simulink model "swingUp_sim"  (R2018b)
settings: Solver=ode4  StartTime=0.0  StopTime=T+Tstb  FixedStep=1e-3  MaxStep=1e-3  RelTol=1e-3  AbsTol=1e-6
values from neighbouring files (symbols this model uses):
  b_0 = (bp_0 + bn_0) / 2    [mainSkript_provedeniSimulaceSwingUp.m]    (also in mainSkript_rovniceSystemu.m = (params.bp_0 + params.bn_0) / 2; mainSkript_overeniRovnic.m = 0; mainSkript_simulaceLQG.m = (bn_0 + bp_0) / 2; mainSkript_LQGexperiment.m = (bn_0 + bp_0) / 2)
  b_1 = params.b_1    [mainSkript_provedeniSimulaceSwingUp.m]    (also in mainSkript_rovniceSystemu.m; mainSkript_overeniRovnic.m; mainSkript_kyvadlaNajednouOdhad.m; mainSkript_simulaceLQG.m)
  b_2 = params.b_2    [mainSkript_provedeniSimulaceSwingUp.m]    (also in mainSkript_rovniceSystemu.m; mainSkript_overeniRovnic.m; mainSkript_kyvadlaNajednouOdhad.m; mainSkript_simulaceLQG.m)
  g = 9.81    [mainSkript_provedeniSimulaceSwingUp.m]    (also in mainSkript_rovniceSystemu.m; mainSkript_overeniRovnic.m; mainSkript_estimaceVozik.m; mainSkript_odhadKyvadlaZvlast.m)
  I_1 = params.I_1    [mainSkript_provedeniSimulaceSwingUp.m]    (also in mainSkript_rovniceSystemu.m; mainSkript_overeniRovnic.m; mainSkript_kyvadlaNajednouOdhad.m; mainSkript_simulaceLQG.m)
  I_2 = params.I_2    [mainSkript_provedeniSimulaceSwingUp.m]    (also in mainSkript_rovniceSystemu.m; mainSkript_overeniRovnic.m; mainSkript_kyvadlaNajednouOdhad.m; mainSkript_simulaceLQG.m)
  K = lqr(sysd, Q_lqr, R_lqr)    [mainSkript_provedeniSimulaceSwingUp.m]    (also in makeFBL.m = [0; -d_2*g*sin(th_1); -d_3*g*sin(th_2)]; mainSkript_simulaceLQG.m = lqr(sysd, Qk, Rk); mainSkript_LQGexperiment.m = lqr(sysd, Q, R); mainSkript_LQGexperiment_integral.m = lqr(sysd, Q, R))
  K1 = [K1(1 : idxL-rez); K1(idxL : idxH); K1(idxH+rez : end)]    [mainSkript_provedeniSimulaceSwingUp.m]
  K2 = [K2(1 : idxL-rez); K2(idxL : idxH); K2(idxH+rez : end)]    [mainSkript_provedeniSimulaceSwingUp.m]
  K3 = [K3(1 : idxL-rez); K3(idxL : idxH); K3(idxH+rez : end)]    [mainSkript_provedeniSimulaceSwingUp.m]
  K4 = [K4(1 : idxL-rez); K4(idxL : idxH); K4(idxH+rez : end)]    [mainSkript_provedeniSimulaceSwingUp.m]
  K5 = [K5(1 : idxL-rez); K5(idxL : idxH); K5(idxH+rez : end)]    [mainSkript_provedeniSimulaceSwingUp.m]
  K6 = [K6(1 : idxL-rez); K6(idxL : idxH); K6(idxH+rez : end)]    [mainSkript_provedeniSimulaceSwingUp.m]
  Ki = [Ki(1 : idxL-rez); Ki(idxL : idxH); Ki(idxH+rez : end)]    [mainSkript_provedeniSimulaceSwingUp.m]
  L_1 = params.L_1    [mainSkript_provedeniSimulaceSwingUp.m]    (also in mainSkript_rovniceSystemu.m; mainSkript_overeniRovnic.m; odhadovane_parametry.m = 0.228; mainSkript_kyvadlaNajednouOdhad.m)
  l_1 = params.l_1    [mainSkript_provedeniSimulaceSwingUp.m]    (also in mainSkript_rovniceSystemu.m; mainSkript_overeniRovnic.m; odhadovane_parametry.m = 0.134; mainSkript_kyvadlaNajednouOdhad.m)
  l_2 = params.l_2    [mainSkript_provedeniSimulaceSwingUp.m]    (also in mainSkript_rovniceSystemu.m; mainSkript_overeniRovnic.m; odhadovane_parametry.m = 0.112; mainSkript_kyvadlaNajednouOdhad.m)
  m_0 = params.m_0    [mainSkript_provedeniSimulaceSwingUp.m]    (also in mainSkript_rovniceSystemu.m; mainSkript_overeniRovnic.m; mainSkript_simulaceLQG.m; mainSkript_LQGexperiment.m)
  m_1 = params.m_1    [mainSkript_provedeniSimulaceSwingUp.m]    (also in mainSkript_rovniceSystemu.m; mainSkript_overeniRovnic.m; mainSkript_kyvadlaNajednouOdhad.m; mainSkript_simulaceLQG.m)
  m_2 = params.m_2    [mainSkript_provedeniSimulaceSwingUp.m]    (also in mainSkript_rovniceSystemu.m; mainSkript_overeniRovnic.m; mainSkript_kyvadlaNajednouOdhad.m; mainSkript_simulaceLQG.m)
  q_0 = [theta0(1) theta1(1) theta2(1) dtheta0(1) dtheta1(1) dtheta2(1)]    [mainSkript_provedeniSimulaceSwingUp.m]    (also in mainSkript_kyvadlaNajednouOdhad.m = cell(1, k); mainSkript_simulaceLQG.m = [0 th1_0 th2_0 0 dth1_0 dth2_0]; mainSkript_LQGexperiment.m = zeros(6,1); mainSkript_LQGexperiment_integral.m = zeros(6,1))
  Q_stab = diag([0.1 6e-3 6e-3 1.2 0.6 0.6])    [mainSkript_provedeniSimulaceSwingUp.m]
  Q_swing = diag([10 10 10 100 100 100])    [mainSkript_provedeniSimulaceSwingUp.m]
  R_stab = diag([0.1 0.5 0.5])    [mainSkript_provedeniSimulaceSwingUp.m]
  R_swing = diag([1 1 1])    [mainSkript_provedeniSimulaceSwingUp.m]
  t_FB = [t_FB(1 : idxL-rez); t_FB(idxL : idxH); t_FB(idxH+rez : end)]    [mainSkript_provedeniSimulaceSwingUp.m]
  Ts = 1e-3    (= 0.001)    [mainSkript_provedeniSimulaceSwingUp.m]    (also in mainSkript_rovniceSystemu.m; mainSkript_simulaceLQG.m; mainSkript_LQGexperiment.m; mainSkript_LQGexperiment_integral.m)
undefined symbols (not defined in the file or in its folder): DiscIntNeverNeededParam
libraries: simulink x5, sharedTrackingLibrary x1
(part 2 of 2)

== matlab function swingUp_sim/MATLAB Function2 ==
function dx = PohybovaRceDIP_basic(y, u, g, m_0, m_1, m_2, I_1, I_2, l_1, l_2, L_1, b_0, b_1, b_2)
%PohybovaRceDIP_basic: Pohybova rovnice dvojiteho kyvadla

dx = zeros(6, 1); % definovani sloupcoveho vektoru derivaci stavu 

dx(1) = conj(y(4)); 
dx(2) = conj(y(5)); 
dx(3) = conj(y(6)); 
dx(4) = conj(y(6))*((b_2*(L_1^2*l_2*m_2^2*cos(y(3)) + I_1*l_2*m_2*cos(y(3)) - L_1^2*l_2*m_2^2*cos(y(2) - y(3))*cos(y(2)) + l_1^2*l_2*m_1*m_2*cos(y(3)) - L_1*l_1*l_2*m_1*m_2*cos(y(2) - y(3))*cos(y(2))))/(I_2*L_1^2*m_2^2 + I_2*l_1^2*m_1^2 + I_1*l_2^2*m_2^2 + I_1*I_2*m_0 + I_1*I_2*m_1 + I_1*I_2*m_2 + L_1^2*l_2^2*m_2^3 + L_1^2*l_2^2*m_0*m_2^2 + L_1^2*l_2^2*m_1*m_2^2 - L_1^2*l_2^2*m_2^3*cos(y(2) - y(3))^2 + I_2*L_1^2*m_0*m_2 + I_2*L_1^2*m_1*m_2 + l_1^2*l_2^2*m_1*m_2^2 + l_1^2*l_2^2*m_1^2*m_2 + I_2*l_1^2*m_0*m_1 + I_1*l_2^2*m_0*m_2 + I_1*l_2^2*m_1*m_2 + I_2*l_1^2*m_1*m_2 - I_2*L_1^2*m_2^2*cos(y(2))^2 - I_2*l_1^2*m_1^2*cos(y(2))^2 - I_1*l_2^2*m_2^2*cos(y(3))^2 - L_1^2*l_2^2*m_2^3*cos(y(2))^2 - L_1^2*l_2^2*m_2^3*cos(y(3))^2 + l_1^2*l_2^2*m_0*m_1*m_2 - l_1^2*l_2^2*m_1^2*m_2*cos(y(2))^2 - l_1^2*l_2^2*m_1*m_2^2*cos(y(3))^2 - L_1^2*l_2^2*m_0*m_2^2*cos(y(2) - y(3))^2 - L_1^2*l_2^2*m_1*m_2^2*cos(y(2) - y(3))^2 - 2*L_1*l_1*l_2^2*m_1*m_2^2*cos(y(2))^2 + 2*L_1^2*l_2^2*m_2^3*cos(y(2) - y(3))*cos(y(2))*cos(y(3)) - 2*I_2*L_1*l_1*m_1*m_2*cos(y(2))^2 + 2*L_1*l_1*l_2^2*m_1*m_2^2*cos(y(2) - y(3))*cos(y(2))*cos(y(3))) - ((b_2 - L_1*l_2*m_2*sin(y(2) - y(3))*y(6))*(L_1*l_2^2*m_2^2*cos(y(2)) + I_2*L_1*m_2*cos(y(2)) + I_2*l_1*m_1*cos(y(2)) - L_1*l_2^2*m_2^2*cos(y(2) - y(3))*cos(y(3)) + l_1*l_2^2*m_1*m_2*cos(y(2))))/(I_2*L_1^2*m_2^2 + I_2*l_1^2*m_1^2 + I_1*l_2^2*m_2^2 + I_1*I_2*m_0 + I_1*I_2*m_1 + I_1*I_2*m_2 + L_1^2*l_2^2*m_2^3 + L_1^2*l_2^2*m_0*m_2^2 + L_1^2*l_2^2*m_1*m_2^2 - L_1^2*l_2^2*m_2^3*cos(y(2) - y(3))^2 + I_2*L_1^2*m_0*m_2 + I_2*L_1^2*m_1*m_2 + l_1^2*l_2^2*m_1*m_2^2 + l_1^2*l_2^2*m_1^2*m_2 + I_2*l_1^2*m_0*m_1 + I_1*l_2^2*m_0*m_2 + I_1*l_2^2*m_1*m_2 + I_2*l_1^2*m_1*m_2 - I_2*L_1^2*m_2^2*cos(y(2))^2 - I_2*l_1^2*m_1^2*cos(y(2))^2 - I_1*l_2^2*m_2^2*cos(y(3))^2 - L_1^2*l_2^2*m_2^3*cos(y(2))^2 - L_1^2*l_2^2*m_2^3*cos(y(3))^2 + l_1^2*l_2^2*m_0*m_1*m_2 - l_1^2*l_2^2*m_1^2*m_2*cos(y(2))^2 - l_1^2*l_2^2*m_1*m_2^2*cos(y(3))^2 - L_1^2*l_2^2*m_0*m_2^2*cos(y(2) - y(3))^2 - L_1^2*l_2^2*m_1*m_2^2*cos(y(2) - y(3))^2 - 2*L_1*l_1*l_2^2*m_1*m_2^2*cos(y(2))^2 + 2*L_1^2*l_2^2*m_2^3*cos(y(2) - y(3))*cos(y(2))*cos(y(3)) - 2*I_2*L_1*l_1*m_1*m_2*cos(y(2))^2 + 2*L_1*l_1*l_2^2*m_1*m_2^2*cos(y(2) - y(3))*cos(y(2))*cos(y(3))) + (l_2*m_2*y(6)*sin(y(3))*(I_1*I_2 + L_1^2*l_2^2*m_2^2 + I_2*L_1^2*m_2 + I_2*l_1^2*m_1 + I_1*l_2^2*m_2 - L_1^2*l_2^2*m_2^2*cos(y(2) - y(3))^2 + l_1^2*l_2^2*m_1*m_2))/(I_2*L_1^2*m_2^2 + I_2*l_1^2*m_1^2 + I_1*l_2^2*m_2^2 + I_1*I_2*m_0 + I_1*I_2*m_1 + I_1*I_2*m_2 + L_1^2*l_2^2*m_2^3 + L_1^2*l_2^2*m_0*m_2^2 + L_1^2*l_2^2*m_1*m_2^2 - L_1^2*l_2^2*m_2^3*cos(y(2) - y(3))^2 + I_2*L_1^2*m_0*m_2 + I_2*L_1^2*m_1*m_2 + l_1^2*l_2^2*m_1*m_2^2 + l_1^2*l_2^2*m_1^2*m_2 + I_2*l_1^2*m_0*m_1 + I_1*l_2^2*m_0*m_2 + I_1*l_2^2*m_1*m_2 + I_2*l_1^2*m_1*m_2 - I_2*L_1^2*m_2^2*cos(y(2))^2 - I_2*l_1^2*m_1^2*cos(y(2))^2 - I_1*l_2^2*m_2^2*cos(y(3))^2 - L_1^2*l_2^2*m_2^3*cos(y(2))^2 - L_1^2*l_2^2*m_2^3*cos(y(3))^2 + l_1^2*l_2^2*m_0*m_1*m_2 - l_1^2*l_2^2*m_1^2*m_2*cos(y(2))^2 - l_1^2*l_2^2*m_1*m_2^2*cos(y(3))^2 - L_1^2*l_2^2*m_0*m_2^2*cos(y(2) - y(3))^2 - L_1^2*l_2^2*m_1*m_2^2*cos(y(2) - y(3))^2 - 2*L_1*l_1*l_2^2*m_1*m_2^2*cos(y(2))^2 + 2*L_1^2*l_2^2*m_2^3*cos(y(2) - y(3))*cos(y(2))*cos(y(3)) - 2*I_2*L_1*l_1*m_1*m_2*cos(y(2))^2 + 2*L_1*l_1*l_2^2*m_1*m_2^2*cos(y(2) - y(3))*cos(y(2))*cos(y(3)))) + conj(y(5))*(((b_1 + b_2)*(L_1*l_2^2*m_2^2*cos(y(2)) + I_2*L_1*m_2*cos(y(2)) + I_2*l_1*m_1*cos(y(2)) - L_1*l_2^2*m_2^2*cos(y(2) - y(3))*cos(y(3)) + l_1*l_2^2*m_1*m_2*cos(y(2))))/(I_2*L_1^2*m_2^2 + I_2*l_1^2*m_1^2 + I_1*l_2^2*m_2^2 + I_1*I_2*m_0 + I_1*I_2*m_1 + I_1*I_2*m_2 + L_1^2*l_2^2*m_2^3 + L_1^2*l_2^2*m_0*m_2^2 + L_1^2*l_2^2*m_1*m_2^2 - L_1^2*l_2^2*m_2^3*cos(y(2) - y(3))^2 + I_2*L_1^2*m_0*m_2 + I_2*L_1^2*m_1*m_2 + l_1^2*l_2^2*m_1*m_2^2 + l_1^2*l_2^2*m_1^2*m_2 + I_2*l_1^2*m_0*m_1 + I_1*l_2^2*m_0*m_2 + I_1*l_2^2*m_1*m_2 + I_2*l_1^2*m_1*m_2 - I_2*L_1^2*m_2^2*cos(y(2))^2 - I_2*l_1^2*m_1^2*cos(y(2))^2 - I_1*l_2^2*m_2^2*cos(y(3))^2 - L_1^2*l_2^2*m_2^3*cos(y(2))^2 - L_1^2*l_2^2*m_2^3*cos(y(3))^2 + l_1^2*l_2^2*m_0*m_1*m_2 - l_1^2*l_2^2*m_1^2*m_2*cos(y(2))^2 - l_1^2*l_2^2*m_1*m_2^2*cos(y(3))^2 - L_1^2*l_2^2*m_0*m_2^2*cos(y(2) - y(3))^2 - L_1^2*l_2^2*m_1*m_2^2*cos(y(2) - y(3))^2 - 2*L_1*l_1*l_2^2*m_1*m_2^2*cos(y(2))^2 + 2*L_1^2*l_2^2*m_2^3*cos(y(2) - y(3))*cos(y(2))*cos(y(3)) - 2*I_2*L_1*l_1*m_1*m_2*cos(y(2))^2 + 2*L_1*l_1*l_2^2*m_1*m_2^2*cos(y(2) - y(3))*cos(y(2))*cos(y(3))) - ((b_2 + L_1*l_2*m_2*sin(y(2) - y(3))*y(5))*(L_1^2*l_2*m_2^2*cos(y(3)) + I_1*l_2*m_2*cos(y(3)) - L_1^2*l_2*m_2^2*cos(y(2) - y(3))*cos(y(2)) + l_1^2*l_2*m_1*m_2*cos(y(3)) - L_1*l_1*l_2*m_1*m_2*cos(y(2) - y(3))*cos(y(2))))/(I_2*L_1^2*m_2^2 + I_2*l_1^2*m_1^2 + I_1*l_2^2*m_2^2 + I_1*I_2*m_0 + I_1*I_2*m_1 + I_1*I_2*m_2 + L_1^2*l_2^2*m_2^3 + L_1^2*l_2^2*m_0*m_2^2 + L_1^2*l_2^2*m_1*m_2^2 - L_1^2*l_2^2*m_2^3*cos(y(2) - y(3))^2 + I_2*L_1^2*m_0*m_2 + I_2*L_1^2*m_1*m_2 + l_1^2*l_2^2*m_1*m_2^2 + l_1^2*l_2^2*m_1^2*m_2 + I_2*l_1^2*m_0*m_1 + I_1*l_2^2*m_0*m_2 + I_1*l_2^2*m_1*m_2 + I_2*l_1^2*m_1*m_2 - I_2*L_1^2*m_2^2*cos(y(2))^2 - I_2*l_1^2*m_1^2*cos(y(2))^2 - I_1*l_2^2*m_2^2*cos(y(3))^2 - L_1^2*l_2^2*m_2^3*cos(y(2))^2 - L_1^2*l_2^2*m_2^3*cos(y(3))^2 + l_1^2*l_2^2*m_0*m_1*m_2 - l_1^2*l_2^2*m_1^2*m_2*cos(y(2))^2 - l_1^2*l_2^2*m_1*m_2^2*cos(y(3))^2 - L_1^2*l_2^2*m_0*m_2^2*cos(y(2) - y(3))^2 - L_1^2*l_2^2*m_1*m_2^2*cos(y(2) - y(3))^2 - 2*L_1*l_1*l_2^2*m_1*m_2^2*cos(y(2))^2 + 2*L_1^2*l_2^2*m_2^3*cos(y(2) - y(3))*cos(y(2))*cos(y(3)) - 2*I_2*L_1*l_1*m_1*m_2*cos(y(2))^2 + 2*L_1*l_1*l_2^2*m_1*m_2^2*cos(y(2) - y(3))*cos(y(2))*cos(y(3))) + (y(5)*sin(y(2))*(L_1*m_2 + l_1*m_1)*(I_1*I_2 + L_1^2*l_2^2*m_2^2 + I_2*L_1^2*m_2 + I_2*l_1^2*m_1 + I_1*l_2^2*m_2 - L_1^2*l_2^2*m_2^2*cos(y(2) - y(3))^2 + l_1^2*l_2^2*m_1*m_2))/(I_2*L_1^2*m_2^2 + I_2*l_1^2*m_1^2 + I_1*l_2^2*m_2^2 + I_1*I_2*m_0 + I_1*I_2*m_1 + I_1*I_2*m_2 + L_1^2*l_2^2*m_2^3 + L_1^2*l_2^2*m_0*m_2^2 + L_1^2*l_2^2*m_1*m_2^2 - L_1^2*l_2^2*m_2^3*cos(y(2) - y(3))^2 + I_2*L_1^2*m_0*m_2 + I_2*L_1^2*m_1*m_2 + l_1^2*l_2^2*m_1*m_2^2 + l_1^2*l_2^2*m_1^2*m_2 + I_2*l_1^2*m_0*m_1 + I_1*l_2^2*m_0*m_2 + I_1*l_2^2*m_1*m_2 + I_2*l_1^2*m_1*m_2 - I_2*L_1^2*m_2^2*cos(y(2))^2 - I_2*l_1^2*m_1^2*cos(y(2))^2 - I_1*l_2^2*m_2^2*cos(y(3))^2 - L_1^2*l_2^2*m_2^3*cos(y(2))^2 - L_1^2*l_2^2*m_2^3*cos(y(3))^2 + l_1^2*l_2^2*m_0*m_1*m_2 - l_1^2*l_2^2*m_1^2*m_2*cos(y(2))^2 - l_1^2*l_2^2*m_1*m_2^2*cos(y(3))^2 - L_1^2*l_2^2*m_0*m_2^2*cos(y(2) - y(3))^2 - L_1^2*l_2^2*m_1*m_2^2*cos(y(2) - y(3))^2 - 2*L_1*l_1*l_2^2*m_1*m_2^2*cos(y(2))^2 + 2*L_1^2*l_2^2*m_2^3*cos(y(2) - y(3))*cos(y(2))*cos(y(3)) - 2*I_2*L_1*l_1*m_1*m_2*cos(y(2))^2 + 2*L_1*l_1*l_2^2*m_1*m_2^2*cos(y(2) - y(3))*cos(y(2))*cos(y(3)))) + (u*(I_1*I_2 + L_1^2*l_2^2*m_2^2 + I_2*L_1^2*m_2 + I_2*l_1^2*m_1 + I_1*l_2^2*m_2 - L_1^2*l_2^2*m_2^2*cos(y(2) - y(3))^2 + l_1^2*l_2^2*m_1*m_2))/(I_2*L_1^2*m_2^2 + I_2*l_1^2*m_1^2 + I_1*l_2^2*m_2^2 + I_1*I_2*m_0 + I_1*I_2*m_1 + I_1*I_2*m_2 + L_1^2*l_2^2*m_2^3 + L_1^2*l_2^2*m_0*m_2^2 + L_1^2*l_2^2*m_1*m_2^2 - L_1^2*l_2^2*m_2^3*cos(y(2) - y(3))^2 + I_2*L_1^2*m_0*m_2 + I_2*L_1^2*m_1*m_2 + l_1^2*l_2^2*m_1*m_2^2 + l_1^2*l_2^2*m_1^2*m_2 + I_2*l_1^2*m_0*m_1 + I_1*l_2^2*m_0*m_2 + I_1*l_2^2*m_1*m_2 + I_2*l_1^2*m_1*m_2 - I_2*L_1^2*m_2^2*cos(y(2))^2 - I_2*l_1^2*m_1^2*cos(y(2))^2 - I_1*l_2^2*m_2^2*cos(y(3))^2 - L_1^2*l_2^2*m_2^3*cos(y(2))^2 - L_1^2*l_2^2*m_2^3*cos(y(3))^2 + l_1^2*l_2^2*m_0*m_1*m_2 - l_1^2*l_2^2*m_1^2*m_2*cos(y(2))^2 - l_1^2*l_2^2*m_1*m_2^2*cos(y(3))^2 - L_1^2*l_2^2*m_0*m_2^2*cos(y(2) - y(3))^2 - L_1^2*l_2^2*m_1*m_2^2*cos(y(2) - y(3))^2 - 2*L_1*l_1*l_2^2*m_1*m_2^2*cos(y(2))^2 + 2*L_1^2*l_2^2*m_2^3*cos(y(2) - y(3))*cos(y(2))*cos(y(3)) - 2*I_2*L_1*l_1*m_1*m_2*cos(y(2))^2 + 2*L_1*l_1*l_2^2*m_1*m_2^2*cos(y(2) - y(3))*cos(y(2))*cos(y(3))) - (b_0*conj(y(4))*(I_1*I_2 + L_1^2*l_2^2*m_2^2 + I_2*L_1^2*m_2 + I_2*l_1^2*m_1 + I_1*l_2^2*m_2 - L_1^2*l_2^2*m_2^2*cos(y(2) - y(3))^2 + l_1^2*l_2^2*m_1*m_2))/(I_2*L_1^2*m_2^2 + I_2*l_1^2*m_1^2 + I_1*l_2^2*m_2^2 + I_1*I_2*m_0 + I_1*I_2*m_1 + I_1*I_2*m_2 + L_1^2*l_2^2*m_2^3 + L_1^2*l_2^2*m_0*m_2^2 + L_1^2*l_2^2*m_1*m_2^2 - L_1^2*l_2^2*m_2^3*cos(y(2) - y(3))^2 + I_2*L_1^2*m_0*m_2 + I_2*L_1^2*m_1*m_2 + l_1^2*l_2^2*m_1*m_2^2 + l_1^2*l_2^2*m_1^2*m_2 + I_2*l_1^2*m_0*m_1 + I_1*l_2^2*m_0*m_2 + I_1*l_2^2*m_1*m_2 + I_2*l_1^2*m_1*m_2 - I_2*L_1^2*m_2^2*cos(y(2))^2 - I_2*l_1^2*m_1^2*cos(y(2))^2 - I_1*l_2^2*m_2^2*cos(y(3))^2 - L_1^2*l_2^2*m_2^3*cos(y(2))^2 - L_1^2*l_2^2*m_2^3*cos(y(3))^2 + l_1^2*l_2^2*m_0*m_1*m_2 - l_1^2*l_2^2*m_1^2*m_2*cos(y(2))^2 - l_1^2*l_2^2*m_1*m_2^2*cos(y(3))^2 - L_1^2*l_2^2*m_0*m_2^2*cos(y(2) - y(3))^2 - L_1^2*l_2^2*m_1*m_2^2*cos(y(2) - y(3))^2 - 2*L_1*l_1*l_2^2*m_1*m_2^2*cos(y(2))^2 + 2*L_1^2*l_2^2*m_2^3*cos(y(2) - y(3))*cos(y(2))*cos(y(3)) - 2*I_2*L_1*l_1*m_1*m_2*cos(y(2))^2 + 2*L_1*l_1*l_2^2*m_1*m_2^2*cos(y(2) - y(3))*cos(y(2))*cos(y(3))) - (g*sin(y(2))*(L_1*m_2 + l_1*m_1)*(L_1*l_2^2*m_2^2*cos(y(2)) + I_2*L_1*m_2*cos(y(2)) + I_2*l_1*m_1*cos(y(2)) - L_1*l_2^2*m_2^2*cos(y(2) - y(3))*cos(y(3)) + l_1*l_2^2*m_1*m_2*cos(y(2))))/(I_2*L_1^2*m_2^2 + I_2*l_1^2*m_1^2 + I_1*l_2^2*m_2^2 + I_1*I_2*m_0 + I_1*I_2*m_1 + I_1*I_2*m_2 + L_1^2*l_2^2*m_2^3 + L_1^2*l_2^2*m_0*m_2^2 + L_1^2*l_2^2*m_1*m_2^2 - L_1^2*l_2^2*m_2^3*cos(y(2) - y(3))^2 + I_2*L_1^2*m_0*m_2 + I_2*L_1^2*m_1*m_2 + l_1^2*l_2^2*m_1*m_2^2 + l_1^2*l_2^2*m_1^2*m_2 + I_2*l_1^2*m_0*m_1 + I_1*l_2^2*m_0*m_2 + I_1*l_2^2*m_1*m_2 + I_2*l_1^2*m_1*m_2 - I_2*L_1^2*m_2^2*cos(y(2))^2 - I_2*l_1^2*m_1^2*cos(y(2))^2 - I_1*l_2^2*m_2^2*cos(y(3))^2 - L_1^2*l_2^2*m_2^3*cos(y(2))^2 - L_1^2*l_2^2*m_2^3*cos(y(3))^2 + l_1^2*l_2^2*m_0*m_1*m_2 - l_1^2*l_2^2*m_1^2*m_2*cos(y(2))^2 - l_1^2*l_2^2*m_1*m_2^2*cos(y(3))^2 - L_1^2*l_2^2*m_0*m_2^2*cos(y(2) - y(3))^2 - L_1^2*l_2^2*m_1*m_2^2*cos(y(2) - y(3))^2 - 2*L_1*l_1*l_2^2*m_1*m_2^2*cos(y(2))^2 + 2*L_1^2*l_2^2*m_2^3*cos(y(2) - y(3))*cos(y(2))*cos(y(3)) - 2*I_2*L_1*l_1*m_1*m_2*cos(y(2))^2 + 2*L_1*l_1*l_2^2*m_1*m_2^2*cos(y(2) - y(3))*cos(y(2))*cos(y(3))) - (g*l_2*m_2*sin(y(3))*(L_1^2*l_2*m_2^2*cos(y(3)) + I_1*l_2*m_2*cos(y(3)) - L_1^2*l_2*m_2^2*cos(y(2) - y(3))*cos(y(2)) + l_1^2*l_2*m_1*m_2*cos(y(3)) - L_1*l_1*l_2*m_1*m_2*cos(y(2) - y(3))*cos(y(2))))/(I_2*L_1^2*m_2^2 + I_2*l_1^2*m_1^2 + I_1*l_2^2*m_2^2 + I_1*I_2*m_0 + I_1*I_2*m_1 + I_1*I_2*m_2 + L_1^2*l_2^2*m_2^3 + L_1^2*l_2^2*m_0*m_2^2 + L_1^2*l_2^2*m_1*m_2^2 - L_1^2*l_2^2*m_2^3*cos(y(2) - y(3))^2 + I_2*L_1^2*m_0*m_2 + I_2*L_1^2*m_1*m_2 + l_1^2*l_2^2*m_1*m_2^2 + l_1^2*l_2^2*m_1^2*m_2 + I_2*l_1^2*m_0*m_1 + I_1*l_2^2*m_0*m_2 + I_1*l_2^2*m_1*m_2 + I_2*l_1^2*m_1*m_2 - I_2*L_1^2*m_2^2*cos(y(2))^2 - I_2*l_1^2*m_1^2*cos(y(2))^2 - I_1*l_2^2*m_2^2*cos(y(3))^2 - L_1^2*l_2^2*m_2^3*cos(y(2))^2 - L_1^2*l_2^2*m_2^3*cos(y(3))^2 + l_1^2*l_2^2*m_0*m_1*m_2 - l_1^2*l_2^2*m_1^2*m_2*cos(y(2))^2 - l_1^2*l_2^2*m_1*m_2^2*cos(y(3))^2 - L_1^2*l_2^2*m_0*m_2^2*cos(y(2) - y(3))^2 - L_1^2*l_2^2*m_1*m_2^2*cos(y(2) - y(3))^2 - 2*L_1*l_1*l_2^2*m_1*m_2^2*cos(y(2))^2 + 2*L_1^2*l_2^2*m_2^3*cos(y(2) - y(3))*cos(y(2))*cos(y(3)) - 2*I_2*L_1*l_1*m_1*m_2*cos(y(2))^2 + 2*L_1*l_1*l_2^2*m_1*m_2^2*cos(y(2) - y(3))*cos(y(2))*cos(y(3))); 
dx(5) = conj(y(6))*((b_2*(L_1*l_2*m_2^2*cos(y(2) - y(3)) + L_1*l_2*m_0*m_2*cos(y(2) - y(3)) + L_1*l_2*m_1*m_2*cos(y(2) - y(3)) - L_1*l_2*m_2^2*cos(y(2))*cos(y(3)) - l_1*l_2*m_1*m_2*cos(y(2))*cos(y(3))))/(I_2*L_1^2*m_2^2 + I_2*l_1^2*m_1^2 + I_1*l_2^2*m_2^2 + I_1*I_2*m_0 + I_1*I_2*m_1 + I_1*I_2*m_2 + L_1^2*l_2^2*m_2^3 + L_1^2*l_2^2*m_0*m_2^2 + L_1^2*l_2^2*m_1*m_2^2 - L_1^2*l_2^2*m_2^3*cos(y(2) - y(3))^2 + I_2*L_1^2*m_0*m_2 + I_2*L_1^2*m_1*m_2 + l_1^2*l_2^2*m_1*m_2^2 + l_1^2*l_2^2*m_1^2*m_2 + I_2*l_1^2*m_0*m_1 + I_1*l_2^2*m_0*m_2 + I_1*l_2^2*m_1*m_2 + I_2*l_1^2*m_1*m_2 - I_2*L_1^2*m_2^2*cos(y(2))^2 - I_2*l_1^2*m_1^2*cos(y(2))^2 - I_1*l_2^2*m_2^2*cos(y(3))^2 - L_1^2*l_2^2*m_2^3*cos(y(2))^2 - L_1^2*l_2^2*m_2^3*cos(y(3))^2 + l_1^2*l_2^2*m_0*m_1*m_2 - l_1^2*l_2^2*m_1^2*m_2*cos(y(2))^2 - l_1^2*l_2^2*m_1*m_2^2*cos(y(3))^2 - L_1^2*l_2^2*m_0*m_2^2*cos(y(2) - y(3))^2 - L_1^2*l_2^2*m_1*m_2^2*cos(y(2) - y(3))^2 - 2*L_1*l_1*l_2^2*m_1*m_2^2*cos(y(2))^2 + 2*L_1^2*l_2^2*m_2^3*cos(y(2) - y(3))*cos(y(2))*cos(y(3)) - 2*I_2*L_1*l_1*m_1*m_2*cos(y(2))^2 + 2*L_1*l_1*l_2^2*m_1*m_2^2*cos(y(2) - y(3))*cos(y(2))*cos(y(3))) + ((b_2 - L_1*l_2*m_2*sin(y(2) - y(3))*y(6))*(I_2*m_0 + I_2*m_1 + I_2*m_2 + l_2^2*m_2^2 + l_2^2*m_0*m_2 + l_2^2*m_1*m_2 - l_2^2*m_2^2*cos(y(3))^2))/(I_2*L_1^2*m_2^2 + I_2*l_1^2*m_1^2 + I_1*l_2^2*m_2^2 + I_1*I_2*m_0 + I_1*I_2*m_1 + I_1*I_2*m_2 + L_1^2*l_2^2*m_2^3 + L_1^2*l_2^2*m_0*m_2^2 + L_1^2*l_2^2*m_1*m_2^2 - L_1^2*l_2^2*m_2^3*cos(y(2) - y(3))^2 + I_2*L_1^2*m_0*m_2 + I_2*L_1^2*m_1*m_2 + l_1^2*l_2^2*m_1*m_2^2 + l_1^2*l_2^2*m_1^2*m_2 + I_2*l_1^2*m_0*m_1 + I_1*l_2^2*m_0*m_2 + I_1*l_2^2*m_1*m_2 + I_2*l_1^2*m_1*m_2 - I_2*L_1^2*m_2^2*cos(y(2))^2 - I_2*l_1^2*m_1^2*cos(y(2))^2 - I_1*l_2^2*m_2^2*cos(y(3))^2 - L_1^2*l_2^2*m_2^3*cos(y(2))^2 - L_1^2*l_2^2*m_2^3*cos(y(3))^2 + l_1^2*l_2^2*m_0*m_1*m_2 - l_1^2*l_2^2*m_1^2*m_2*cos(y(2))^2 - l_1^2*l_2^2*m_1*m_2^2*cos(y(3))^2 - L_1^2*l_2^2*m_0*m_2^2*cos(y(2) - y(3))^2 - L_1^2*l_2^2*m_1*m_2^2*cos(y(2) - y(3))^2 - 2*L_1*l_1*l_2^2*m_1*m_2^2*cos(y(2))^2 + 2*L_1^2*l_2^2*m_2^3*cos(y(2) - y(3))*cos(y(2))*cos(y(3)) - 2*I_2*L_1*l_1*m_1*m_2*cos(y(2))^2 + 2*L_1*l_1*l_2^2*m_1*m_2^2*cos(y(2) - y(3))*cos(y(2))*cos(y(3))) - (l_2*m_2*y(6)*sin(y(3))*(L_1*l_2^2*m_2^2*cos(y(2)) + I_2*L_1*m_2*cos(y(2)) + I_2*l_1*m_1*cos(y(2)) - L_1*l_2^2*m_2^2*cos(y(2) - y(3))*cos(y(3)) + l_1*l_2^2*m_1*m_2*cos(y(2))))/(I_2*L_1^2*m_2^2 + I_2*l_1^2*m_1^2 + I_1*l_2^2*m_2^2 + I_1*I_2*m_0 + I_1*I_2*m_1 + I_1*I_2*m_2 + L_1^2*l_2^2*m_2^3 + L_1^2*l_2^2*m_0*m_2^2 + L_1^2*l_2^2*m_1*m_2^2 - L_1^2*l_2^2*m_2^3*cos(y(2) - y(3))^2 + I_2*L_1^2*m_0*m_2 + I_2*L_1^2*m_1*m_2 + l_1^2*l_2^2*m_1*m_2^2 + l_1^2*l_2^2*m_1^2*m_2 + I_2*l_1^2*m_0*m_1 + I_1*l_2^2*m_0*m_2 + I_1*l_2^2*m_1*m_2 + I_2*l_1^2*m_1*m_2 - I_2*L_1^2*m_2^2*cos(y(2))^2 - I_2*l_1^2*m_1^2*cos(y(2))^2 - I_1*l_2^2*m_2^2*cos(y(3))^2 - L_1^2*l_2^2*m_2^3*cos(y(2))^2 - L_1^2*l_2^2*m_2^3*cos(y(3))^2 + l_1^2*l_2^2*m_0*m_1*m_2 - l_1^2*l_2^2*m_1^2*m_2*cos(y(2))^2 - l_1^2*l_2^2*m_1*m_2^2*cos(y(3))^2 - L_1^2*l_2^2*m_0*m_2^2*cos(y(2) - y(3))^2 - L_1^2*l_2^2*m_1*m_2^2*cos(y(2) - y(3))^2 - 2*L_1*l_1*l_2^2*m_1*m_2^2*cos(y(2))^2 + 2*L_1^2*l_2^2*m_2^3*cos(y(2) - y(3))*cos(y(2))*cos(y(3)) - 2*I_2*L_1*l_1*m_1*m_2*cos(y(2))^2 + 2*L_1*l_1*l_2^2*m_1*m_2^2*cos(y(2) - y(3))*cos(y(2))*cos(y(3)))) - conj(y(5))*(((b_1 + b_2)*(I_2*m_0 + I_2*m_1 + I_2*m_2 + l_2^2*m_2^2 + l_2^2*m_0*m_2 + l_2^2*m_1*m_2 - l_2^2*m_2^2*cos(y(3))^2))/(I_2*L_1^2*m_2^2 + I_2*l_1^2*m_1^2 + I_1*l_2^2*m_2^2 + I_1*I_2*m_0 + I_1*I_2*m_1 + I_1*I_2*m_2 + L_1^2*l_2^2*m_2^3 + L_1^2*l_2^2*m_0*m_2^2 + L_1^2*l_2^2*m_1*m_2^2 - L_1^2*l_2^2*m_2^3*cos(y(2) - y(3))^2 + I_2*L_1^2*m_0*m_2 + I_2*L_1^2*m_1*m_2 + l_1^2*l_2^2*m_1*m_2^2 + l_1^2*l_2^2*m_1^2*m_2 + I_2*l_1^2*m_0*m_1 + I_1*l_2^2*m_0*m_2 + I_1*l_2^2*m_1*m_2 + I_2*l_1^2*m_1*m_2 - I_2*L_1^2*m_2^2*cos(y(2))^2 - I_2*l_1^2*m_1^2*cos(y(2))^2 - I_1*l_2^2*m_2^2*cos(y(3))^2 - L_1^2*l_2^2*m_2^3*cos(y(2))^2 - L_1^2*l_2^2*m_2^3*cos(y(3))^2 + l_1^2*l_2^2*m_0*m_1*m_2 - l_1^2*l_2^2*m_1^2*m_2*cos(y(2))^2 - l_1^2*l_2^2*m_1*m_2^2*cos(y(3))^2 - L_1^2*l_2^2*m_0*m_2^2*cos(y(2) - y(3))^2 - L_1^2*l_2^2*m_1*m_2^2*cos(y(2) - y(3))^2 - 2*L_1*l_1*l_2^2*m_1*m_2^2*cos(y(2))^2 + 2*L_1^2*l_2^2*m_2^3*cos(y(2) - y(3))*cos(y(2))*cos(y(3)) - 2*I_2*L_1*l_1*m_1*m_2*cos(y(2))^2 + 2*L_1*l_1*l_2^2*m_1*m_2^2*cos(y(2) - y(3))*cos(y(2))*cos(y(3))) + ((b_2 + L_1*l_2*m_2*sin(y(2) - y(3))*y(5))*(L_1*l_2*m_2^2*cos(y(2) - y(3)) + L_1*l_2*m_0*m_2*cos(y(2) - y(3)) + L_1*l_2*m_1*m_2*cos(y(2) - y(3)) - L_1*l_2*m_2^2*cos(y(2))*cos(y(3)) - l_1*l_2*m_1*m_2*cos(y(2))*cos(y(3))))/(I_2*L_1^2*m_2^2 + I_2*l_1^2*m_1^2 + I_1*l_2^2*m_2^2 + I_1*I_2*m_0 + I_1*I_2*m_1 + I_1*I_2*m_2 + L_1^2*l_2^2*m_2^3 + L_1^2*l_2^2*m_0*m_2^2 + L_1^2*l_2^2*m_1*m_2^2 - L_1^2*l_2^2*m_2^3*cos(y(2) - y(3))^2 + I_2*L_1^2*m_0*m_2 + I_2*L_1^2*m_1*m_2 + l_1^2*l_2^2*m_1*m_2^2 + l_1^2*l_2^2*m_1^2*m_2 + I_2*l_1^2*m_0*m_1 + I_1*l_2^2*m_0*m_2 + I_1*l_2^2*m_1*m_2 + I_2*l_1^2*m_1*m_2 - I_2*L_1^2*m_2^2*cos(y(2))^2 - I_2*l_1^2*m_1^2*cos(y(2))^2 - I_1*l_2^2*m_2^2*cos(y(3))^2 - L_1^2*l_2^2*m_2^3*cos(y(2))^2 - L_1^2*l_2^2*m_2^3*cos(y(3))^2 + l_1^2*l_2^2*m_0*m_1*m_2 - l_1^2*l_2^2*m_1^2*m_2*cos(y(2))^2 - l_1^2*l_2^2*m_1*m_2^2*cos(y(3))^2 - L_1^2*l_2^2*m_0*m_2^2*cos(y(2) - y(3))^2 - L_1^2*l_2^2*m_1*m_2^2*cos(y(2) - y(3))^2 - 2*L_1*l_1*l_2^2*m_1*m_2^2*cos(y(2))^2 + 2*L_1^2*l_2^2*m_2^3*cos(y(2) - y(3))*cos(y(2))*cos(y(3)) - 2*I_2*L_1*l_1*m_1*m_2*cos(y(2))^2 + 2*L_1*l_1*l_2^2*m_1*m_2^2*cos(y(2) - y(3))*cos(y(2))*cos(y(3))) + (y(5)*sin(y(2))*(L_1*m_2 + l_1*m_1)*(L_1*l_2^2*m_2^2*cos(y(2)) + I_2*L_1*m_2*cos(y(2)) + I_2*l_1*m_1*cos(y(2)) - L_1*l_2^2*m_2^2*cos(y(2) - y(3))*cos(y(3)) + l_1*l_2^2*m_1*m_2*cos(y(2))))/(I_2*L_1^2*m_2^2 + I_2*l_1^2*m_1^2 + I_1*l_2^2*m_2^2 + I_1*I_2*m_0 + I_1*I_2*m_1 + I_1*I_2*m_2 + L_1^2*l_2^2*m_2^3 + L_1^2*l_2^2*m_0*m_2^2 + L_1^2*l_2^2*m_1*m_2^2 - L_1^2*l_2^2*m_2^3*cos(y(2) - y(3))^2 + I_2*L_1^2*m_0*m_2 + I_2*L_1^2*m_1*m_2 + l_1^2*l_2^2*m_1*m_2^2 + l_1^2*l_2^2*m_1^2*m_2 + I_2*l_1^2*m_0*m_1 + I_1*l_2^2*m_0*m_2 + I_1*l_2^2*m_1*m_2 + I_2*l_1^2*m_1*m_2 - I_2*L_1^2*m_2^2*cos(y(2))^2 - I_2*l_1^2*m_1^2*cos(y(2))^2 - I_1*l_2^2*m_2^2*cos(y(3))^2 - L_1^2*l_2^2*m_2^3*cos(y(2))^2 - L_1^2*l_2^2*m_2^3*cos(y(3))^2 + l_1^2*l_2^2*m_0*m_1*m_2 - l_1^2*l_2^2*m_1^2*m_2*cos(y(2))^2 - l_1^2*l_2^2*m_1*m_2^2*cos(y(3))^2 - L_1^2*l_2^2*m_0*m_2^2*cos(y(2) - y(3))^2 - L_1^2*l_2^2*m_1*m_2^2*cos(y(2) - y(3))^2 - 2*L_1*l_1*l_2^2*m_1*m_2^2*cos(y(2))^2 + 2*L_1^2*l_2^2*m_2^3*cos(y(2) - y(3))*cos(y(2))*cos(y(3)) - 2*I_2*L_1*l_1*m_1*m_2*cos(y(2))^2 + 2*L_1*l_1*l_2^2*m_1*m_2^2*cos(y(2) - y(3))*cos(y(2))*cos(y(3)))) - (u*(L_1*l_2^2*m_2^2*cos(y(2)) + I_2*L_1*m_2*cos(y(2)) + I_2*l_1*m_1*cos(y(2)) - L_1*l_2^2*m_2^2*cos(y(2) - y(3))*cos(y(3)) + l_1*l_2^2*m_1*m_2*cos(y(2))))/(I_2*L_1^2*m_2^2 + I_2*l_1^2*m_1^2 + I_1*l_2^2*m_2^2 + I_1*I_2*m_0 + I_1*I_2*m_1 + I_1*I_2*m_2 + L_1^2*l_2^2*m_2^3 + L_1^2*l_2^2*m_0*m_2^2 + L_1^2*l_2^2*m_1*m_2^2 - L_1^2*l_2^2*m_2^3*cos(y(2) - y(3))^2 + I_2*L_1^2*m_0*m_2 + I_2*L_1^2*m_1*m_2 + l_1^2*l_2^2*m_1*m_2^2 + l_1^2*l_2^2*m_1^2*m_2 + I_2*l_1^2*m_0*m_1 + I_1*l_2^2*m_0*m_2 + I_1*l_2^2*m_1*m_2 + I_2*l_1^2*m_1*m_2 - I_2*L_1^2*m_2^2*cos(y(2))^2 - I_2*l_1^2*m_1^2*cos(y(2))^2 - I_1*l_2^2*m_2^2*cos(y(3))^2 - L_1^2*l_2^2*m_2^3*cos(y(2))^2 - L_1^2*l_2^2*m_2^3*cos(y(3))^2 + l_1^2*l_2^2*m_0*m_1*m_2 - l_1^2*l_2^2*m_1^2*m_2*cos(y(2))^2 - l_1^2*l_2^2*m_1*m_2^2*cos(y(3))^2 - L_1^2*l_2^2*m_0*m_2^2*cos(y(2) - y(3))^2 - L_1^2*l_2^2*m_1*m_2^2*cos(y(2) - y(3))^2 - 2*L_1*l_1*l_2^2*m_1*m_2^2*cos(y(2))^2 + 2*L_1^2*l_2^2*m_2^3*cos(y(2) - y(3))*cos(y(2))*cos(y(3)) - 2*I_2*L_1*l_1*m_1*m_2*cos(y(2))^2 + 2*L_1*l_1*l_2^2*m_1*m_2^2*cos(y(2) - y(3))*cos(y(2))*cos(y(3))) + (b_0*conj(y(4))*(L_1*l_2^2*m_2^2*cos(y(2)) + I_2*L_1*m_2*cos(y(2)) + I_2*l_1*m_1*cos(y(2)) - L_1*l_2^2*m_2^2*cos(y(2) - y(3))*cos(y(3)) + l_1*l_2^2*m_1*m_2*cos(y(2))))/(I_2*L_1^2*m_2^2 + I_2*l_1^2*m_1^2 + I_1*l_2^2*m_2^2 + I_1*I_2*m_0 + I_1*I_2*m_1 + I_1*I_2*m_2 + L_1^2*l_2^2*m_2^3 + L_1^2*l_2^2*m_0*m_2^2 + L_1^2*l_2^2*m_1*m_2^2 - L_1^2*l_2^2*m_2^3*cos(y(2) - y(3))^2 + I_2*L_1^2*m_0*m_2 + I_2*L_1^2*m_1*m_2 + l_1^2*l_2^2*m_1*m_2^2 + l_1^2*l_2^2*m_1^2*m_2 + I_2*l_1^2*m_0*m_1 + I_1*l_2^2*m_0*m_2 + I_1*l_2^2*m_1*m_2 + I_2*l_1^2*m_1*m_2 - I_2*L_1^2*m_2^2*cos(y(2))^2 - I_2*l_1^2*m_1^2*cos(y(2))^2 - I_1*l_2^2*m_2^2*cos(y(3))^2 - L_1^2*l_2^2*m_2^3*cos(y(2))^2 - L_1^2*l_2^2*m_2^3*cos(y(3))^2 + l_1^2*l_2^2*m_0*m_1*m_2 - l_1^2*l_2^2*m_1^2*m_2*cos(y(2))^2 - l_1^2*l_2^2*m_1*m_2^2*cos(y(3))^2 - L_1^2*l_2^2*m_0*m_2^2*cos(y(2) - y(3))^2 - L_1^2*l_2^2*m_1*m_2^2*cos(y(2) - y(3))^2 - 2*L_1*l_1*l_2^2*m_1*m_2^2*cos(y(2))^2 + 2*L_1^2*l_2^2*m_2^3*cos(y(2) - y(3))*cos(y(2))*cos(y(3)) - 2*I_2*L_1*l_1*m_1*m_2*cos(y(2))^2 + 2*L_1*l_1*l_2^2*m_1*m_2^2*cos(y(2) - y(3))*cos(y(2))*cos(y(3))) + (g*sin(y(2))*(L_1*m_2 + l_1*m_1)*(I_2*m_0 + I_2*m_1 + I_2*m_2 + l_2^2*m_2^2 + l_2^2*m_0*m_2 + l_2^2*m_1*m_2 - l_2^2*m_2^2*cos(y(3))^2))/(I_2*L_1^2*m_2^2 + I_2*l_1^2*m_1^2 + I_1*l_2^2*m_2^2 + I_1*I_2*m_0 + I_1*I_2*m_1 + I_1*I_2*m_2 + L_1^2*l_2^2*m_2^3 + L_1^2*l_2^2*m_0*m_2^2 + L_1^2*l_2^2*m_1*m_2^2 - L_1^2*l_2^2*m_2^3*cos(y(2) - y(3))^2 + I_2*L_1^2*m_0*m_2 + I_2*L_1^2*m_1*m_2 + l_1^2*l_2^2*m_1*m_2^2 + l_1^2*l_2^2*m_1^2*m_2 + I_2*l_1^2*m_0*m_1 + I_1*l_2^2*m_0*m_2 + I_1*l_2^2*m_1*m_2 + I_2*l_1^2*m_1*m_2 - I_2*L_1^2*m_2^2*cos(y(2))^2 - I_2*l_1^2*m_1^2*cos(y(2))^2 - I_1*l_2^2*m_2^2*cos(y(3))^2 - L_1^2*l_2^2*m_2^3*cos(y(2))^2 - L_1^2*l_2^2*m_2^3*cos(y(3))^2 + l_1^2*l_2^2*m_0*m_1*m_2 - l_1^2*l_2^2*m_1^2*m_2*cos(y(2))^2 - l_1^2*l_2^2*m_1*m_2^2*cos(y(3))^2 - L_1^2*l_2^2*m_0*m_2^2*cos(y(2) - y(3))^2 - L_1^2*l_2^2*m_1*m_2^2*cos(y(2) - y(3))^2 - 2*L_1*l_1*l_2^2*m_1*m_2^2*cos(y(2))^2 + 2*L_1^2*l_2^2*m_2^3*cos(y(2) - y(3))*cos(y(2))*cos(y(3)) - 2*I_2*L_1*l_1*m_1*m_2*cos(y(2))^2 + 2*L_1*l_1*l_2^2*m_1*m_2^2*cos(y(2) - y(3))*cos(y(2))*cos(y(3))) - (g*l_2*m_2*sin(y(3))*(L_1*l_2*m_2^2*cos(y(2) - y(3)) + L_1*l_2*m_0*m_2*cos(y(2) - y(3)) + L_1*l_2*m_1*m_2*cos(y(2) - y(3)) - L_1*l_2*m_2^2*cos(y(2))*cos(y(3)) - l_1*l_2*m_1*m_2*cos(y(2))*cos(y(3))))/(I_2*L_1^2*m_2^2 + I_2*l_1^2*m_1^2 + I_1*l_2^2*m_2^2 + I_1*I_2*m_0 + I_1*I_2*m_1 + I_1*I_2*m_2 + L_1^2*l_2^2*m_2^3 + L_1^2*l_2^2*m_0*m_2^2 + L_1^2*l_2^2*m_1*m_2^2 - L_1^2*l_2^2*m_2^3*cos(y(2) - y(3))^2 + I_2*L_1^2*m_0*m_2 + I_2*L_1^2*m_1*m_2 + l_1^2*l_2^2*m_1*m_2^2 + l_1^2*l_2^2*m_1^2*m_2 + I_2*l_1^2*m_0*m_1 + I_1*l_2^2*m_0*m_2 + I_1*l_2^2*m_1*m_2 + I_2*l_1^2*m_1*m_2 - I_2*L_1^2*m_2^2*cos(y(2))^2 - I_2*l_1^2*m_1^2*cos(y(2))^2 - I_1*l_2^2*m_2^2*cos(y(3))^2 - L_1^2*l_2^2*m_2^3*cos(y(2))^2 - L_1^2*l_2^2*m_2^3*cos(y(3))^2 + l_1^2*l_2^2*m_0*m_1*m_2 - l_1^2*l_2^2*m_1^2*m_2*cos(y(2))^2 - l_1^2*l_2^2*m_1*m_2^2*cos(y(3))^2 - L_1^2*l_2^2*m_0*m_2^2*cos(y(2) - y(3))^2 - L_1^2*l_2^2*m_1*m_2^2*cos(y(2) - y(3))^2 - 2*L_1*l_1*l_2^2*m_1*m_2^2*cos(y(2))^2 + 2*L_1^2*l_2^2*m_2^3*cos(y(2) - y(3))*cos(y(2))*cos(y(3)) - 2*I_2*L_1*l_1*m_1*m_2*cos(y(2))^2 + 2*L_1*l_1*l_2^2*m_1*m_2^2*cos(y(2) - y(3))*cos(y(2))*cos(y(3))); 
dx(6) = conj(y(5))*(((b_1 + b_2)*(L_1*l_2*m_2^2*cos(y(2) - y(3)) + L_1*l_2*m_0*m_2*cos(y(2) - y(3)) + L_1*l_2*m_1*m_2*cos(y(2) - y(3)) - L_1*l_2*m_2^2*cos(y(2))*cos(y(3)) - l_1*l_2*m_1*m_2*cos(y(2))*cos(y(3))))/(I_2*L_1^2*m_2^2 + I_2*l_1^2*m_1^2 + I_1*l_2^2*m_2^2 + I_1*I_2*m_0 + I_1*I_2*m_1 + I_1*I_2*m_2 + L_1^2*l_2^2*m_2^3 + L_1^2*l_2^2*m_0*m_2^2 + L_1^2*l_2^2*m_1*m_2^2 - L_1^2*l_2^2*m_2^3*cos(y(2) - y(3))^2 + I_2*L_1^2*m_0*m_2 + I_2*L_1^2*m_1*m_2 + l_1^2*l_2^2*m_1*m_2^2 + l_1^2*l_2^2*m_1^2*m_2 + I_2*l_1^2*m_0*m_1 + I_1*l_2^2*m_0*m_2 + I_1*l_2^2*m_1*m_2 + I_2*l_1^2*m_1*m_2 - I_2*L_1^2*m_2^2*cos(y(2))^2 - I_2*l_1^2*m_1^2*cos(y(2))^2 - I_1*l_2^2*m_2^2*cos(y(3))^2 - L_1^2*l_2^2*m_2^3*cos(y(2))^2 - L_1^2*l_2^2*m_2^3*cos(y(3))^2 + l_1^2*l_2^2*m_0*m_1*m_2 - l_1^2*l_2^2*m_1^2*m_2*cos(y(2))^2 - l_1^2*l_2^2*m_1*m_2^2*cos(y(3))^2 - L_1^2*l_2^2*m_0*m_2^2*cos(y(2) - y(3))^2 - L_1^2*l_2^2*m_1*m_2^2*cos(y(2) - y(3))^2 - 2*L_1*l_1*l_2^2*m_1*m_2^2*cos(y(2))^2 + 2*L_1^2*l_2^2*m_2^3*cos(y(2) - y(3))*cos(y(2))*cos(y(3)) - 2*I_2*L_1*l_1*m_1*m_2*cos(y(2))^2 + 2*L_1*l_1*l_2^2*m_1*m_2^2*cos(y(2) - y(3))*cos(y(2))*cos(y(3))) + ((b_2 + L_1*l_2*m_2*sin(y(2) - y(3))*y(5))*(I_1*m_0 + I_1*m_1 + I_1*m_2 + L_1^2*m_2^2 + l_1^2*m_1^2 + l_1^2*m_0*m_1 + l_1^2*m_1*m_2 - L_1^2*m_2^2*cos(y(2))^2 - l_1^2*m_1^2*cos(y(2))^2 + L_1^2*m_0*m_2 + L_1^2*m_1*m_2 - 2*L_1*l_1*m_1*m_2*cos(y(2))^2))/(I_2*L_1^2*m_2^2 + I_2*l_1^2*m_1^2 + I_1*l_2^2*m_2^2 + I_1*I_2*m_0 + I_1*I_2*m_1 + I_1*I_2*m_2 + L_1^2*l_2^2*m_2^3 + L_1^2*l_2^2*m_0*m_2^2 + L_1^2*l_2^2*m_1*m_2^2 - L_1^2*l_2^2*m_2^3*cos(y(2) - y(3))^2 + I_2*L_1^2*m_0*m_2 + I_2*L_1^2*m_1*m_2 + l_1^2*l_2^2*m_1*m_2^2 + l_1^2*l_2^2*m_1^2*m_2 + I_2*l_1^2*m_0*m_1 + I_1*l_2^2*m_0*m_2 + I_1*l_2^2*m_1*m_2 + I_2*l_1^2*m_1*m_2 - I_2*L_1^2*m_2^2*cos(y(2))^2 - I_2*l_1^2*m_1^2*cos(y(2))^2 - I_1*l_2^2*m_2^2*cos(y(3))^2 - L_1^2*l_2^2*m_2^3*cos(y(2))^2 - L_1^2*l_2^2*m_2^3*cos(y(3))^2 + l_1^2*l_2^2*m_0*m_1*m_2 - l_1^2*l_2^2*m_1^2*m_2*cos(y(2))^2 - l_1^2*l_2^2*m_1*m_2^2*cos(y(3))^2 - L_1^2*l_2^2*m_0*m_2^2*cos(y(2) - y(3))^2 - L_1^2*l_2^2*m_1*m_2^2*cos(y(2) - y(3))^2 - 2*L_1*l_1*l_2^2*m_1*m_2^2*cos(y(2))^2 + 2*L_1^2*l_2^2*m_2^3*cos(y(2) - y(3))*cos(y(2))*cos(y(3)) - 2*I_2*L_1*l_1*m_1*m_2*cos(y(2))^2 + 2*L_1*l_1*l_2^2*m_1*m_2^2*cos(y(2) - y(3))*cos(y(2))*cos(y(3))) - (y(5)*sin(y(2))*(L_1*m_2 + l_1*m_1)*(L_1^2*l_2*m_2^2*cos(y(3)) + I_1*l_2*m_2*cos(y(3)) - L_1^2*l_2*m_2^2*cos(y(2) - y(3))*cos(y(2)) + l_1^2*l_2*m_1*m_2*cos(y(3)) - L_1*l_1*l_2*m_1*m_2*cos(y(2) - y(3))*cos(y(2))))/(I_2*L_1^2*m_2^2 + I_2*l_1^2*m_1^2 + I_1*l_2^2*m_2^2 + I_1*I_2*m_0 + I_1*I_2*m_1 + I_1*I_2*m_2 + L_1^2*l_2^2*m_2^3 + L_1^2*l_2^2*m_0*m_2^2 + L_1^2*l_2^2*m_1*m_2^2 - L_1^2*l_2^2*m_2^3*cos(y(2) - y(3))^2 + I_2*L_1^2*m_0*m_2 + I_2*L_1^2*m_1*m_2 + l_1^2*l_2^2*m_1*m_2^2 + l_1^2*l_2^2*m_1^2*m_2 + I_2*l_1^2*m_0*m_1 + I_1*l_2^2*m_0*m_2 + I_1*l_2^2*m_1*m_2 + I_2*l_1^2*m_1*m_2 - I_2*L_1^2*m_2^2*cos(y(2))^2 - I_2*l_1^2*m_1^2*cos(y(2))^2 - I_1*l_2^2*m_2^2*cos(y(3))^2 - L_1^2*l_2^2*m_2^3*cos(y(2))^2 - L_1^2*l_2^2*m_2^3*cos(y(3))^2 + l_1^2*l_2^2*m_0*m_1*m_2 - l_1^2*l_2^2*m_1^2*m_2*cos(y(2))^2 - l_1^2*l_2^2*m_1*m_2^2*cos(y(3))^2 - L_1^2*l_2^2*m_0*m_2^2*cos(y(2) - y(3))^2 - L_1^2*l_2^2*m_1*m_2^2*cos(y(2) - y(3))^2 - 2*L_1*l_1*l_2^2*m_1*m_2^2*cos(y(2))^2 + 2*L_1^2*l_2^2*m_2^3*cos(y(2) - y(3))*cos(y(2))*cos(y(3)) - 2*I_2*L_1*l_1*m_1*m_2*cos(y(2))^2 + 2*L_1*l_1*l_2^2*m_1*m_2^2*cos(y(2) - y(3))*cos(y(2))*cos(y(3)))) - conj(y(6))*((b_2*(I_1*m_0 + I_1*m_1 + I_1*m_2 + L_1^2*m_2^2 + l_1^2*m_1^2 + l_1^2*m_0*m_1 + l_1^2*m_1*m_2 - L_1^2*m_2^2*cos(y(2))^2 - l_1^2*m_1^2*cos(y(2))^2 + L_1^2*m_0*m_2 + L_1^2*m_1*m_2 - 2*L_1*l_1*m_1*m_2*cos(y(2))^2))/(I_2*L_1^2*m_2^2 + I_2*l_1^2*m_1^2 + I_1*l_2^2*m_2^2 + I_1*I_2*m_0 + I_1*I_2*m_1 + I_1*I_2*m_2 + L_1^2*l_2^2*m_2^3 + L_1^2*l_2^2*m_0*m_2^2 + L_1^2*l_2^2*m_1*m_2^2 - L_1^2*l_2^2*m_2^3*cos(y(2) - y(3))^2 + I_2*L_1^2*m_0*m_2 + I_2*L_1^2*m_1*m_2 + l_1^2*l_2^2*m_1*m_2^2 + l_1^2*l_2^2*m_1^2*m_2 + I_2*l_1^2*m_0*m_1 + I_1*l_2^2*m_0*m_2 + I_1*l_2^2*m_1*m_2 + I_2*l_1^2*m_1*m_2 - I_2*L_1^2*m_2^2*cos(y(2))^2 - I_2*l_1^2*m_1^2*cos(y(2))^2 - I_1*l_2^2*m_2^2*cos(y(3))^2 - L_1^2*l_2^2*m_2^3*cos(y(2))^2 - L_1^2*l_2^2*m_2^3*cos(y(3))^2 + l_1^2*l_2^2*m_0*m_1*m_2 - l_1^2*l_2^2*m_1^2*m_2*cos(y(2))^2 - l_1^2*l_2^2*m_1*m_2^2*cos(y(3))^2 - L_1^2*l_2^2*m_0*m_2^2*cos(y(2) - y(3))^2 - L_1^2*l_2^2*m_1*m_2^2*cos(y(2) - y(3))^2 - 2*L_1*l_1*l_2^2*m_1*m_2^2*cos(y(2))^2 + 2*L_1^2*l_2^2*m_2^3*cos(y(2) - y(3))*cos(y(2))*cos(y(3)) - 2*I_2*L_1*l_1*m_1*m_2*cos(y(2))^2 + 2*L_1*l_1*l_2^2*m_1*m_2^2*cos(y(2) - y(3))*cos(y(2))*cos(y(3))) + ((b_2 - L_1*l_2*m_2*sin(y(2) - y(3))*y(6))*(L_1*l_2*m_2^2*cos(y(2) - y(3)) + L_1*l_2*m_0*m_2*cos(y(2) - y(3)) + L_1*l_2*m_1*m_2*cos(y(2) - y(3)) - L_1*l_2*m_2^2*cos(y(2))*cos(y(3)) - l_1*l_2*m_1*m_2*cos(y(2))*cos(y(3))))/(I_2*L_1^2*m_2^2 + I_2*l_1^2*m_1^2 + I_1*l_2^2*m_2^2 + I_1*I_2*m_0 + I_1*I_2*m_1 + I_1*I_2*m_2 + L_1^2*l_2^2*m_2^3 + L_1^2*l_2^2*m_0*m_2^2 + L_1^2*l_2^2*m_1*m_2^2 - L_1^2*l_2^2*m_2^3*cos(y(2) - y(3))^2 + I_2*L_1^2*m_0*m_2 + I_2*L_1^2*m_1*m_2 + l_1^2*l_2^2*m_1*m_2^2 + l_1^2*l_2^2*m_1^2*m_2 + I_2*l_1^2*m_0*m_1 + I_1*l_2^2*m_0*m_2 + I_1*l_2^2*m_1*m_2 + I_2*l_1^2*m_1*m_2 - I_2*L_1^2*m_2^2*cos(y(2))^2 - I_2*l_1^2*m_1^2*cos(y(2))^2 - I_1*l_2^2*m_2^2*cos(y(3))^2 - L_1^2*l_2^2*m_2^3*cos(y(2))^2 - L_1^2*l_2^2*m_2^3*cos(y(3))^2 + l_1^2*l_2^2*m_0*m_1*m_2 - l_1^2*l_2^2*m_1^2*m_2*cos(y(2))^2 - l_1^2*l_2^2*m_1*m_2^2*cos(y(3))^2 - L_1^2*l_2^2*m_0*m_2^2*cos(y(2) - y(3))^2 - L_1^2*l_2^2*m_1*m_2^2*cos(y(2) - y(3))^2 - 2*L_1*l_1*l_2^2*m_1*m_2^2*cos(y(2))^2 + 2*L_1^2*l_2^2*m_2^3*cos(y(2) - y(3))*cos(y(2))*cos(y(3)) - 2*I_2*L_1*l_1*m_1*m_2*cos(y(2))^2 + 2*L_1*l_1*l_2^2*m_1*m_2^2*cos(y(2) - y(3))*cos(y(2))*cos(y(3))) + (l_2*m_2*y(6)*sin(y(3))*(L_1^2*l_2*m_2^2*cos(y(3)) + I_1*l_2*m_2*cos(y(3)) - L_1^2*l_2*m_2^2*cos(y(2) - y(3))*cos(y(2)) + l_1^2*l_2*m_1*m_2*cos(y(3)) - L_1*l_1*l_2*m_1*m_2*cos(y(2) - y(3))*cos(y(2))))/(I_2*L_1^2*m_2^2 + I_2*l_1^2*m_1^2 + I_1*l_2^2*m_2^2 + I_1*I_2*m_0 + I_1*I_2*m_1 + I_1*I_2*m_2 + L_1^2*l_2^2*m_2^3 + L_1^2*l_2^2*m_0*m_2^2 + L_1^2*l_2^2*m_1*m_2^2 - L_1^2*l_2^2*m_2^3*cos(y(2) - y(3))^2 + I_2*L_1^2*m_0*m_2 + I_2*L_1^2*m_1*m_2 + l_1^2*l_2^2*m_1*m_2^2 + l_1^2*l_2^2*m_1^2*m_2 + I_2*l_1^2*m_0*m_1 + I_1*l_2^2*m_0*m_2 + I_1*l_2^2*m_1*m_2 + I_2*l_1^2*m_1*m_2 - I_2*L_1^2*m_2^2*cos(y(2))^2 - I_2*l_1^2*m_1^2*cos(y(2))^2 - I_1*l_2^2*m_2^2*cos(y(3))^2 - L_1^2*l_2^2*m_2^3*cos(y(2))^2 - L_1^2*l_2^2*m_2^3*cos(y(3))^2 + l_1^2*l_2^2*m_0*m_1*m_2 - l_1^2*l_2^2*m_1^2*m_2*cos(y(2))^2 - l_1^2*l_2^2*m_1*m_2^2*cos(y(3))^2 - L_1^2*l_2^2*m_0*m_2^2*cos(y(2) - y(3))^2 - L_1^2*l_2^2*m_1*m_2^2*cos(y(2) - y(3))^2 - 2*L_1*l_1*l_2^2*m_1*m_2^2*cos(y(2))^2 + 2*L_1^2*l_2^2*m_2^3*cos(y(2) - y(3))*cos(y(2))*cos(y(3)) - 2*I_2*L_1*l_1*m_1*m_2*cos(y(2))^2 + 2*L_1*l_1*l_2^2*m_1*m_2^2*cos(y(2) - y(3))*cos(y(2))*cos(y(3)))) - (u*(L_1^2*l_2*m_2^2*cos(y(3)) + I_1*l_2*m_2*cos(y(3)) - L_1^2*l_2*m_2^2*cos(y(2) - y(3))*cos(y(2)) + l_1^2*l_2*m_1*m_2*cos(y(3)) - L_1*l_1*l_2*m_1*m_2*cos(y(2) - y(3))*cos(y(2))))/(I_2*L_1^2*m_2^2 + I_2*l_1^2*m_1^2 + I_1*l_2^2*m_2^2 + I_1*I_2*m_0 + I_1*I_2*m_1 + I_1*I_2*m_2 + L_1^2*l_2^2*m_2^3 + L_1^2*l_2^2*m_0*m_2^2 + L_1^2*l_2^2*m_1*m_2^2 - L_1^2*l_2^2*m_2^3*cos(y(2) - y(3))^2 + I_2*L_1^2*m_0*m_2 + I_2*L_1^2*m_1*m_2 + l_1^2*l_2^2*m_1*m_2^2 + l_1^2*l_2^2*m_1^2*m_2 + I_2*l_1^2*m_0*m_1 + I_1*l_2^2*m_0*m_2 + I_1*l_2^2*m_1*m_2 + I_2*l_1^2*m_1*m_2 - I_2*L_1^2*m_2^2*cos(y(2))^2 - I_2*l_1^2*m_1^2*cos(y(2))^2 - I_1*l_2^2*m_2^2*cos(y(3))^2 - L_1^2*l_2^2*m_2^3*cos(y(2))^2 - L_1^2*l_2^2*m_2^3*cos(y(3))^2 + l_1^2*l_2^2*m_0*m_1*m_2 - l_1^2*l_2^2*m_1^2*m_2*cos(y(2))^2 - l_1^2*l_2^2*m_1*m_2^2*cos(y(3))^2 - L_1^2*l_2^2*m_0*m_2^2*cos(y(2) - y(3))^2 - L_1^2*l_2^2*m_1*m_2^2*cos(y(2) - y(3))^2 - 2*L_1*l_1*l_2^2*m_1*m_2^2*cos(y(2))^2 + 2*L_1^2*l_2^2*m_2^3*cos(y(2) - y(3))*cos(y(2))*cos(y(3)) - 2*I_2*L_1*l_1*m_1*m_2*cos(y(2))^2 + 2*L_1*l_1*l_2^2*m_1*m_2^2*cos(y(2) - y(3))*cos(y(2))*cos(y(3))) + (b_0*conj(y(4))*(L_1^2*l_2*m_2^2*cos(y(3)) + I_1*l_2*m_2*cos(y(3)) - L_1^2*l_2*m_2^2*cos(y(2) - y(3))*cos(y(2)) + l_1^2*l_2*m_1*m_2*cos(y(3)) - L_1*l_1*l_2*m_1*m_2*cos(y(2) - y(3))*cos(y(2))))/(I_2*L_1^2*m_2^2 + I_2*l_1^2*m_1^2 + I_1*l_2^2*m_2^2 + I_1*I_2*m_0 + I_1*I_2*m_1 + I_1*I_2*m_2 + L_1^2*l_2^2*m_2^3 + L_1^2*l_2^2*m_0*m_2^2 + L_1^2*l_2^2*m_1*m_2^2 - L_1^2*l_2^2*m_2^3*cos(y(2) - y(3))^2 + I_2*L_1^2*m_0*m_2 + I_2*L_1^2*m_1*m_2 + l_1^2*l_2^2*m_1*m_2^2 + l_1^2*l_2^2*m_1^2*m_2 + I_2*l_1^2*m_0*m_1 + I_1*l_2^2*m_0*m_2 + I_1*l_2^2*m_1*m_2 + I_2*l_1^2*m_1*m_2 - I_2*L_1^2*m_2^2*cos(y(2))^2 - I_2*l_1^2*m_1^2*cos(y(2))^2 - I_1*l_2^2*m_2^2*cos(y(3))^2 - L_1^2*l_2^2*m_2^3*cos(y(2))^2 - L_1^2*l_2^2*m_2^3*cos(y(3))^2 + l_1^2*l_2^2*m_0*m_1*m_2 - l_1^2*l_2^2*m_1^2*m_2*cos(y(2))^2 - l_1^2*l_2^2*m_1*m_2^2*cos(y(3))^2 - L_1^2*l_2^2*m_0*m_2^2*cos(y(2) - y(3))^2 - L_1^2*l_2^2*m_1*m_2^2*cos(y(2) - y(3))^2 - 2*L_1*l_1*l_2^2*m_1*m_2^2*cos(y(2))^2 + 2*L_1^2*l_2^2*m_2^3*cos(y(2) - y(3))*cos(y(2))*cos(y(3)) - 2*I_2*L_1*l_1*m_1*m_2*cos(y(2))^2 + 2*L_1*l_1*l_2^2*m_1*m_2^2*cos(y(2) - y(3))*cos(y(2))*cos(y(3))) - (g*sin(y(2))*(L_1*m_2 + l_1*m_1)*(L_1*l_2*m_2^2*cos(y(2) - y(3)) + L_1*l_2*m_0*m_2*cos(y(2) - y(3)) + L_1*l_2*m_1*m_2*cos(y(2) - y(3)) - L_1*l_2*m_2^2*cos(y(2))*cos(y(3)) - l_1*l_2*m_1*m_2*cos(y(2))*cos(y(3))))/(I_2*L_1^2*m_2^2 + I_2*l_1^2*m_1^2 + I_1*l_2^2*m_2^2 + I_1*I_2*m_0 + I_1*I_2*m_1 + I_1*I_2*m_2 + L_1^2*l_2^2*m_2^3 + L_1^2*l_2^2*m_0*m_2^2 + L_1^2*l_2^2*m_1*m_2^2 - L_1^2*l_2^2*m_2^3*cos(y(2) - y(3))^2 + I_2*L_1^2*m_0*m_2 + I_2*L_1^2*m_1*m_2 + l_1^2*l_2^2*m_1*m_2^2 + l_1^2*l_2^2*m_1^2*m_2 + I_2*l_1^2*m_0*m_1 + I_1*l_2^2*m_0*m_2 + I_1*l_2^2*m_1*m_2 + I_2*l_1^2*m_1*m_2 - I_2*L_1^2*m_2^2*cos(y(2))^2 - I_2*l_1^2*m_1^2*cos(y(2))^2 - I_1*l_2^2*m_2^2*cos(y(3))^2 - L_1^2*l_2^2*m_2^3*cos(y(2))^2 - L_1^2*l_2^2*m_2^3*cos(y(3))^2 + l_1^2*l_2^2*m_0*m_1*m_2 - l_1^2*l_2^2*m_1^2*m_2*cos(y(2))^2 - l_1^2*l_2^2*m_1*m_2^2*cos(y(3))^2 - L_1^2*l_2^2*m_0*m_2^2*cos(y(2) - y(3))^2 - L_1^2*l_2^2*m_1*m_2^2*cos(y(2) - y(3))^2 - 2*L_1*l_1*l_2^2*m_1*m_2^2*cos(y(2))^2 + 2*L_1^2*l_2^2*m_2^3*cos(y(2) - y(3))*cos(y(2))*cos(y(3)) - 2*I_2*L_1*l_1*m_1*m_2*cos(y(2))^2 + 2*L_1*l_1*l_2^2*m_1*m_2^2*cos(y(2) - y(3))*cos(y(2))*cos(y(3))) + (g*l_2*m_2*sin(y(3))*(I_1*m_0 + I_1*m_1 + I_1*m_2 + L_1^2*m_2^2 + l_1^2*m_1^2 + l_1^2*m_0*m_1 + l_1^2*m_1*m_2 - L_1^2*m_2^2*cos(y(2))^2 - l_1^2*m_1^2*cos(y(2))^2 + L_1^2*m_0*m_2 + L_1^2*m_1*m_2 - 2*L_1*l_1*m_1*m_2*cos(y(2))^2))/(I_2*L_1^2*m_2^2 + I_2*l_1^2*m_1^2 + I_1*l_2^2*m_2^2 + I_1*I_2*m_0 + I_1*I_2*m_1 + I_1*I_2*m_2 + L_1^2*l_2^2*m_2^3 + L_1^2*l_2^2*m_0*m_2^2 + L_1^2*l_2^2*m_1*m_2^2 - L_1^2*l_2^2*m_2^3*cos(y(2) - y(3))^2 + I_2*L_1^2*m_0*m_2 + I_2*L_1^2*m_1*m_2 + l_1^2*l_2^2*m_1*m_2^2 + l_1^2*l_2^2*m_1^2*m_2 + I_2*l_1^2*m_0*m_1 + I_1*l_2^2*m_0*m_2 + I_1*l_2^2*m_1*m_2 + I_2*l_1^2*m_1*m_2 - I_2*L_1^2*m_2^2*cos(y(2))^2 - I_2*l_1^2*m_1^2*cos(y(2))^2 - I_1*l_2^2*m_2^2*cos(y(3))^2 - L_1^2*l_2^2*m_2^3*cos(y(2))^2 - L_1^2*l_2^2*m_2^3*cos(y(3))^2 + l_1^2*l_2^2*m_0*m_1*m_2 - l_1^2*l_2^2*m_1^2*m_2*cos(y(2))^2 - l_1^2*l_2^2*m_1*m_2^2*cos(y(3))^2 - L_1^2*l_2^2*m_0*m_2^2*cos(y(2) - y(3))^2 - L_1^2*l_2^2*m_1*m_2^2*cos(y(2) - y(3))^2 - 2*L_1*l_1*l_2^2*m_1*m_2^2*cos(y(2))^2 + 2*L_1^2*l_2^2*m_2^3*cos(y(2) - y(3))*cos(y(2))*cos(y(3)) - 2*I_2*L_1*l_1*m_1*m_2*cos(y(2))^2 + 2*L_1*l_1*l_2^2*m_1*m_2^2*cos(y(2) - y(3))*cos(y(2))*cos(y(3)));

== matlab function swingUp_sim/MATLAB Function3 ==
function dx = PohybovaRceDIP_simplified(y, u, g, m_1, m_2, I_1, I_2, l_1, l_2, L_1, b_1, b_2)
%PohybovaRceDIP_simplified: Zjednodusena pohybova rovnice dvojiteho kyvadla

dx = zeros(6, 1); % definovani sloupcoveho vektoru derivaci stavu 

dx(1) = conj(y(4)); 
dx(2) = conj(y(5)); 
dx(3) = conj(y(6)); 
dx(4) = u; 
dx(5) = conj(y(6))*(((I_2 + l_2^2*m_2)*(b_2 - L_1*l_2*m_2*sin(y(2) - y(3))*y(6)))/(I_1*I_2 + L_1^2*l_2^2*m_2^2 + I_2*L_1^2*m_2 + I_2*l_1^2*m_1 + I_1*l_2^2*m_2 - L_1^2*l_2^2*m_2^2*cos(y(2) - y(3))^2 + l_1^2*l_2^2*m_1*m_2) + (L_1*b_2*l_2*m_2*cos(y(2) - y(3)))/(I_1*I_2 + L_1^2*l_2^2*m_2^2 + I_2*L_1^2*m_2 + I_2*l_1^2*m_1 + I_1*l_2^2*m_2 - L_1^2*l_2^2*m_2^2*cos(y(2) - y(3))^2 + l_1^2*l_2^2*m_1*m_2)) - conj(y(5))*(((b_1 + b_2)*(I_2 + l_2^2*m_2))/(I_1*I_2 + L_1^2*l_2^2*m_2^2 + I_2*L_1^2*m_2 + I_2*l_1^2*m_1 + I_1*l_2^2*m_2 - L_1^2*l_2^2*m_2^2*cos(y(2) - y(3))^2 + l_1^2*l_2^2*m_1*m_2) + (L_1*l_2*m_2*cos(y(2) - y(3))*(b_2 + L_1*l_2*m_2*sin(y(2) - y(3))*y(5)))/(I_1*I_2 + L_1^2*l_2^2*m_2^2 + I_2*L_1^2*m_2 + I_2*l_1^2*m_1 + I_1*l_2^2*m_2 - L_1^2*l_2^2*m_2^2*cos(y(2) - y(3))^2 + l_1^2*l_2^2*m_1*m_2)) - (u*(L_1*l_2^2*m_2^2*cos(y(2)) + I_2*L_1*m_2*cos(y(2)) + I_2*l_1*m_1*cos(y(2)) - L_1*l_2^2*m_2^2*cos(y(2) - y(3))*cos(y(3)) + l_1*l_2^2*m_1*m_2*cos(y(2))))/(I_1*I_2 + L_1^2*l_2^2*m_2^2 + I_2*L_1^2*m_2 + I_2*l_1^2*m_1 + I_1*l_2^2*m_2 - L_1^2*l_2^2*m_2^2*cos(y(2) - y(3))^2 + l_1^2*l_2^2*m_1*m_2) + (g*sin(y(2))*(I_2 + l_2^2*m_2)*(L_1*m_2 + l_1*m_1))/(I_1*I_2 + L_1^2*l_2^2*m_2^2 + I_2*L_1^2*m_2 + I_2*l_1^2*m_1 + I_1*l_2^2*m_2 - L_1^2*l_2^2*m_2^2*cos(y(2) - y(3))^2 + l_1^2*l_2^2*m_1*m_2) - (L_1*g*l_2^2*m_2^2*cos(y(2) - y(3))*sin(y(3)))/(I_1*I_2 + L_1^2*l_2^2*m_2^2 + I_2*L_1^2*m_2 + I_2*l_1^2*m_1 + I_1*l_2^2*m_2 - L_1^2*l_2^2*m_2^2*cos(y(2) - y(3))^2 + l_1^2*l_2^2*m_1*m_2); 
dx(6) = conj(y(5))*(((b_2 + L_1*l_2*m_2*sin(y(2) - y(3))*y(5))*(I_1 + L_1^2*m_2 + l_1^2*m_1))/(I_1*I_2 + L_1^2*l_2^2*m_2^2 + I_2*L_1^2*m_2 + I_2*l_1^2*m_1 + I_1*l_2^2*m_2 - L_1^2*l_2^2*m_2^2*cos(y(2) - y(3))^2 + l_1^2*l_2^2*m_1*m_2) + (L_1*l_2*m_2*cos(y(2) - y(3))*(b_1 + b_2))/(I_1*I_2 + L_1^2*l_2^2*m_2^2 + I_2*L_1^2*m_2 + I_2*l_1^2*m_1 + I_1*l_2^2*m_2 - L_1^2*l_2^2*m_2^2*cos(y(2) - y(3))^2 + l_1^2*l_2^2*m_1*m_2)) - conj(y(6))*((b_2*(I_1 + L_1^2*m_2 + l_1^2*m_1))/(I_1*I_2 + L_1^2*l_2^2*m_2^2 + I_2*L_1^2*m_2 + I_2*l_1^2*m_1 + I_1*l_2^2*m_2 - L_1^2*l_2^2*m_2^2*cos(y(2) - y(3))^2 + l_1^2*l_2^2*m_1*m_2) + (L_1*l_2*m_2*cos(y(2) - y(3))*(b_2 - L_1*l_2*m_2*sin(y(2) - y(3))*y(6)))/(I_1*I_2 + L_1^2*l_2^2*m_2^2 + I_2*L_1^2*m_2 + I_2*l_1^2*m_1 + I_1*l_2^2*m_2 - L_1^2*l_2^2*m_2^2*cos(y(2) - y(3))^2 + l_1^2*l_2^2*m_1*m_2)) - (u*(L_1^2*l_2*m_2^2*cos(y(3)) + I_1*l_2*m_2*cos(y(3)) - L_1^2*l_2*m_2^2*cos(y(2) - y(3))*cos(y(2)) + l_1^2*l_2*m_1*m_2*cos(y(3)) - L_1*l_1*l_2*m_1*m_2*cos(y(2) - y(3))*cos(y(2))))/(I_1*I_2 + L_1^2*l_2^2*m_2^2 + I_2*L_1^2*m_2 + I_2*l_1^2*m_1 + I_1*l_2^2*m_2 - L_1^2*l_2^2*m_2^2*cos(y(2) - y(3))^2 + l_1^2*l_2^2*m_1*m_2) + (g*l_2*m_2*sin(y(3))*(I_1 + L_1^2*m_2 + l_1^2*m_1))/(I_1*I_2 + L_1^2*l_2^2*m_2^2 + I_2*L_1^2*m_2 + I_2*l_1^2*m_1 + I_1*l_2^2*m_2 - L_1^2*l_2^2*m_2^2*cos(y(2) - y(3))^2 + l_1^2*l_2^2*m_1*m_2) - (L_1*g*l_2*m_2*cos(y(2) - y(3))*sin(y(2))*(L_1*m_2 + l_1*m_1))/(I_1*I_2 + L_1^2*l_2^2*m_2^2 + I_2*L_1^2*m_2 + I_2*l_1^2*m_1 + I_1*l_2^2*m_2 - L_1^2*l_2^2*m_2^2*cos(y(2) - y(3))^2 + l_1^2*l_2^2*m_1*m_2);

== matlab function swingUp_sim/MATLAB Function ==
function u = feedbackLinearization_pn0(y, v)
%feedbackLinearization: castecna feedback linearizace - ziskani vstupu pro nelinearni system

if y(4) >=  0 % pro kladne rychlosti b_0 = bp_0
    
    u = (407227096910748504076914119243960960953492563523831375978747126050092199441462516336971030531937534480482304000000*sin(2*y(3)) - 11500407088910324146229444568754977472486398737404017444437732424056822108965631195323726200028988324684156570173440*sin(2*y(2)) - 26418000604491414037729084897799230433872258733859352182489594880568277844574960151329460006886992568489370189824000*v - 38059545187225181939804639757279163112146715315650517610285758127260518450645593649384707915346925197249740800000000*y(4) + 1172314687962316426730830231269620537460387231131907996374896271565425291433805422561032232418857117704806989824000*v*cos(2*y(2)) - 41511426800280173708146189525378283481497712897434391027395221819581263959374364560343632062378953565798400000000*v*cos(2*y(3)) + 492045723340722615495028011226454017452946366853739292052179612616638111902587083211769291479153157578833218567541*y(5)^2*sin(y(2)) + 50295857773834799189479864038880676635514908862422130557322253979452276518744379794851283378667411165394501632000*y(6)^2*sin(y(3)) + 5356276663601442609699708077417056239453993665034575770751736002464515867882739888144337237499995121254400000000000*v*cos(2*y(2) - 2*y(3)) + 7263050669987173942265987748836687610041066651788929085738879757556545879587283107325219312762880000000000000000*cos(2*y(2) - y(3))*y(5) + 8006247597711649632596918481927449887090166632858331748059638477387765391009508487908250783580160000000000000000000*cos(2*y(2) - 2*y(3))*y(4) - 7263050669987173942265987748836687610041066651788929085738879757556545879587283107325219312762880000000000000000*cos(2*y(2) - y(3))*y(6) + 9598375883327782360522300495416211152969762948065962014481980256228086771971518560933848655035928202444800000000*sin(y(2) - 2*y(3))*y(5)^2 + 22282331604835469067702428897433847264384452559489323601535491529380520538303306109460532984911023308800000000000*y(5)*cos(y(2)) - 6178224845503107713832181816779954459693611170215349909809604911723664888652117385880781865730703360000000000000*y(5)*cos(y(3)) - 9017716265682905405409027352953892971060347895536436742159557775367226695516784382665165340536523980800000000000*y(6)*cos(y(2)) + 6178224845503107713832181816779954459693611170215349909809604911723664888652117385880781865730703360000000000000*y(6)*cos(y(3)) + 64496908227243814717814088608977115510649855854183576524253318118857625462989267473669950699504969770336256000000*y(6)^2*sin(2*y(2) - y(3)) - 4270195300250416688401631268211930494099518640040372875987811061856265168098600038736183951360000000000000000000*cos(y(2) - 2*y(3))*y(5) + 1728158897354997701608804393581124427815894932443086303985916132599091409916404886843173109760000000000000000000*cos(y(2) - 2*y(3))*y(6))/(15845632502852867518708790067200000000*(239006967539396035935973030594274634756909155463627229724502722981906396484375*cos(2*y(2) - 2*y(3)) - 1136174764783351394902810531656107874226455178782169636600620141135272382496583));
    
else % pro zaprone rychlosti b_0 = bn_0
    
    u = (407227096910748504076914119243960960953492563523831375978747126050092199441462516336971030531937534480482304000000*sin(2*y(3)) - 11500407088910324146229444568754977472486398737404017444437732424056822108965631195323726200028988324684156570173440*sin(2*y(2)) - 26418000604491414037729084897799230433872258733859352182489594880568277844574960151329460006886992568489370189824000*v - 52825751718264196288369386446192831394527468905436723885993376191470792027027698283024774260848205320998092800000000*y(4) + 1172314687962316426730830231269620537460387231131907996374896271565425291433805422561032232418857117704806989824000*v*cos(2*y(2)) - 41511426800280173708146189525378283481497712897434391027395221819581263959374364560343632062378953565798400000000*v*cos(2*y(3)) + 492045723340722615495028011226454017452946366853739292052179612616638111902587083211769291479153157578833218567541*y(5)^2*sin(y(2)) + 50295857773834799189479864038880676635514908862422130557322253979452276518744379794851283378667411165394501632000*y(6)^2*sin(y(3)) + 5356276663601442609699708077417056239453993665034575770751736002464515867882739888144337237499995121254400000000000*v*cos(2*y(2) - 2*y(3)) + 7263050669987173942265987748836687610041066651788929085738879757556545879587283107325219312762880000000000000000*cos(2*y(2) - y(3))*y(5) + 11112482971384133026983829878608441058644044285713816069421841210421164855775185351709848827330560000000000000000000*cos(2*y(2) - 2*y(3))*y(4) - 7263050669987173942265987748836687610041066651788929085738879757556545879587283107325219312762880000000000000000*cos(2*y(2) - y(3))*y(6) + 9598375883327782360522300495416211152969762948065962014481980256228086771971518560933848655035928202444800000000*sin(y(2) - 2*y(3))*y(5)^2 + 22282331604835469067702428897433847264384452559489323601535491529380520538303306109460532984911023308800000000000*y(5)*cos(y(2)) - 6178224845503107713832181816779954459693611170215349909809604911723664888652117385880781865730703360000000000000*y(5)*cos(y(3)) - 9017716265682905405409027352953892971060347895536436742159557775367226695516784382665165340536523980800000000000*y(6)*cos(y(2)) + 6178224845503107713832181816779954459693611170215349909809604911723664888652117385880781865730703360000000000000*y(6)*cos(y(3)) + 64496908227243814717814088608977115510649855854183576524253318118857625462989267473669950699504969770336256000000*y(6)^2*sin(2*y(2) - y(3)) - 4270195300250416688401631268211930494099518640040372875987811061856265168098600038736183951360000000000000000000*cos(y(2) - 2*y(3))*y(5) + 1728158897354997701608804393581124427815894932443086303985916132599091409916404886843173109760000000000000000000*cos(y(2) - 2*y(3))*y(6))/(15845632502852867518708790067200000000*(239006967539396035935973030594274634756909155463627229724502722981906396484375*cos(2*y(2) - 2*y(3)) - 1136174764783351394902810531656107874226455178782169636600620141135272382496583));
    
end
